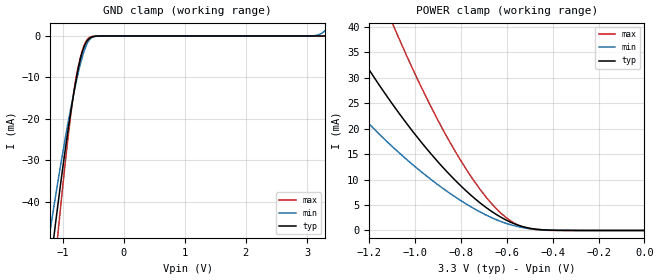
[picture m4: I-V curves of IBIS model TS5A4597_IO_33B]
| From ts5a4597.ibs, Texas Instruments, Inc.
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[Model]   TS5A4597_IO_33B
Model_type  Terminator
| variable   typ   min   max
C_comp   4.78pF   4.11pF   5.54pF
| C_tri-state   4.78pF   4.11pF   5.54pF
[Temperature Range]   40   100   -40
| Ambient temperature   25   85   -40
[Voltage range]   3.3   2.7   3.6
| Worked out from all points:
|   GND clamp passes 1 mA (typ) near -0.59 V on its own axis
|   POWER clamp passes 1 mA (typ) near -0.55 V on its own axis
[GND Clamp]
| TS5A4597_IO_33B
|   Voltage   I(typ)   I(min)   I(max)
-3.3V     -371.9mA   -304.2mA   -447mA
-1.21V    -56.76mA   -47.69mA   -68.49mA
-1.145V   -48.86mA   -41.51mA   -58.32mA
-1.11V    -44.71mA   -38.26mA   -52.97mA
-1.08V    -41.22mA   -35.53mA   -48.45mA
-1.05V    -37.8mA    -32.84mA   -44.02mA
-875mV    -19.33mA   -18.25mA   -20.19mA
-790mV    -11.62mA   -12.02mA   -11.07mA
-670mV    -3.519mA   -4.767mA   -3.273mA
-555mV    -544.2uA   -838.3uA   -337.4uA
3.05V     104.1pA    16.34uA    37.43pA
3.3V      235.7pA    1.349mA    41.17pA
[POWER Clamp]
| TS5A4597_IO_33B
|   Voltage   I(typ)   I(min)   I(max)
-3.3V     260.2mA    185.1mA    385.8mA
-1.555V   59.32mA    39.51mA    96.63mA
-1.315V   39.82mA    26.4mA     65.39mA
-1.095V   24.57mA    16.29mA    40.27mA
-1.075V   23.32mA    15.46mA    38.19mA
-920mV    14.48mA    9.641mA    23.34mA
-810mV    9.171mA    6.137mA    14.4mA
-705mV    5.002mA    3.361mA    7.385mA
-605mV    2.088mA    1.422mA    2.589mA
-550mV    1.024mA    740.6uA    1.04mA
-470mV    238uA      207.2uA    150.2uA
-48.03fV  235.7pA    1.249nA    49.19pA
